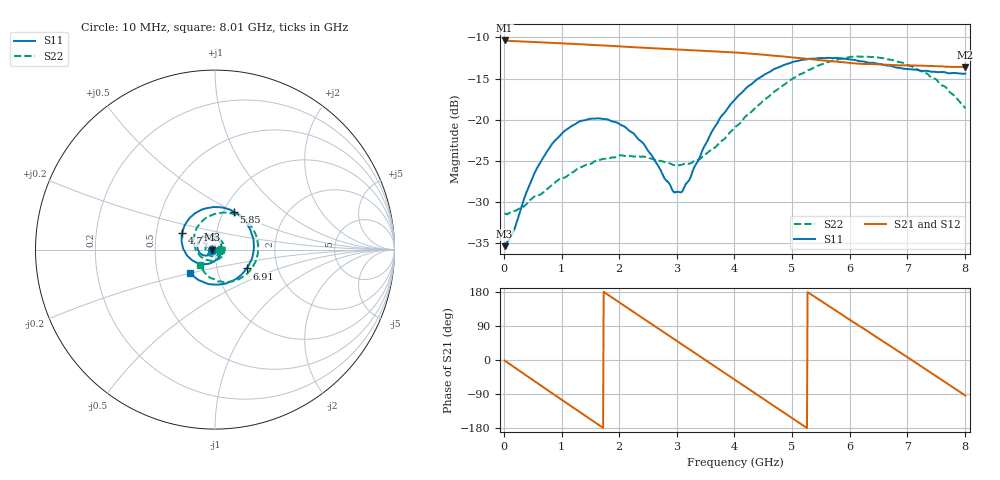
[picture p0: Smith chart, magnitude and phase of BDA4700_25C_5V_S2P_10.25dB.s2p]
!Agilent Technologies,E5071B,MY42404982,A.09.10
!Date: Mon Oct 20 13:31:11 2025
!Data & Calibration Information:
!Freq	S11:SOLT2(ON)	S21:SOLT2(ON)	S12:SOLT2(ON)	S22:SOLT2(ON)
# Hz S RI R 50
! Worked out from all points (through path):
!   801 points, 10 MHz to 8.01 GHz, reference 50 ohm
!   highest |S21| = -10.36 dB at 10 MHz (marker M1); lowest = -13.6 dB at 8 GHz (marker M2)
!   group delay of S21, straight-line fit = 282 ps
!   lowest |S11| = -35.4 dB at 10 MHz (marker M3), VSWR 1.03, Z = 48.3 - j0.118 ohm
!   |S11| at or under -10 dB: start of sweep to end of sweep
!   |S22| runs from -31.5 to -12.3 dB; largest |S21 - S12| = 0.0023
!   S11 on the Smith chart (normalised r, x): 10 MHz: 0.97, -0.00; 4.72 GHz: 0.68, +0.13; 5.85 GHz: 1.12, +0.50; 6.91 GHz: 1.39, -0.30; 8.01 GHz: 0.73, -0.20
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1e7  -0.017 -0.00122  0.3032 -0.00666  0.3032 -0.00685  0.0271 -0.00149
3.3e8  -0.024 -0.0207  0.2446 -0.1714  0.2445 -0.1717  0.022 -0.0196
7.2e8  -0.0521 -0.0335  0.0727 -0.2853  0.0727 -0.2854  -0.00233 -0.0372
1.02e9  -0.0806 -0.0223  -0.0842 -0.2785  -0.0843 -0.2787  -0.0296 -0.0329
1.35e9  -0.0982 0.0102  -0.2231 -0.1811  -0.2232 -0.1811  -0.0515 -0.00482
1.93e9  -0.0639 0.0728  -0.2621 0.0988  -0.2621 0.0987  -0.0246 0.0538
2.32e9  -0.0123 0.0759  -0.1354 0.2395  -0.1354 0.2396  0.0223 0.0557
2.68e9  0.027 0.0447  0.0336 0.2692  0.0337 0.2691  0.0521 0.0212
2.94e9  0.0361 0.00666  0.1483 0.2235  0.1484 0.2231  0.0519 -0.0116
3.08e9  0.0329 -0.0153  0.1981 0.1788  0.1971 0.1794  0.0444 -0.0294
3.53e9  -0.0178 -0.0721  0.2613 -0.0161  0.2615 -0.0166  -0.00932 -0.0623
4.01e9  -0.1148 -0.0666  0.1561 -0.2032  0.1563 -0.203  -0.0821 -0.0364
4.37e9  -0.1735 -0.00224  0.00369 -0.2507  0.00345 -0.251  -0.1164 0.0253
4.72e9  -0.1841 0.091  -0.14 -0.2003  -0.1397 -0.201  -0.1085 0.1045
5.35e9  -0.0584 0.2277  -0.2303 0.0354  -0.2304 0.0348  0.0249 0.2029
5.85e9  0.1049 0.2107  -0.1166 0.1916  -0.1163 0.1916  0.1721 0.1605
6.27e9  0.1985 0.1057  0.037 0.2149  0.0389 0.2143  0.238 0.041
6.68e9  0.2102 -0.0352  0.1666 0.1367  0.1671 0.1365  0.2166 -0.0854
6.91e9  0.1768 -0.1049  0.205 0.0616  0.2053 0.0609  0.1724 -0.1412
7.46e9  0.0202 -0.1947  0.166 -0.132  0.1658 -0.1322  0.0194 -0.1771
8e9  -0.1358 -0.1339  -0.0111 -0.2087  -0.0111 -0.209  -0.0811 -0.0864
8.01e9  -0.138 -0.1319  -0.0148 -0.2085  -0.0145 -0.2087  -0.0821 -0.0839
